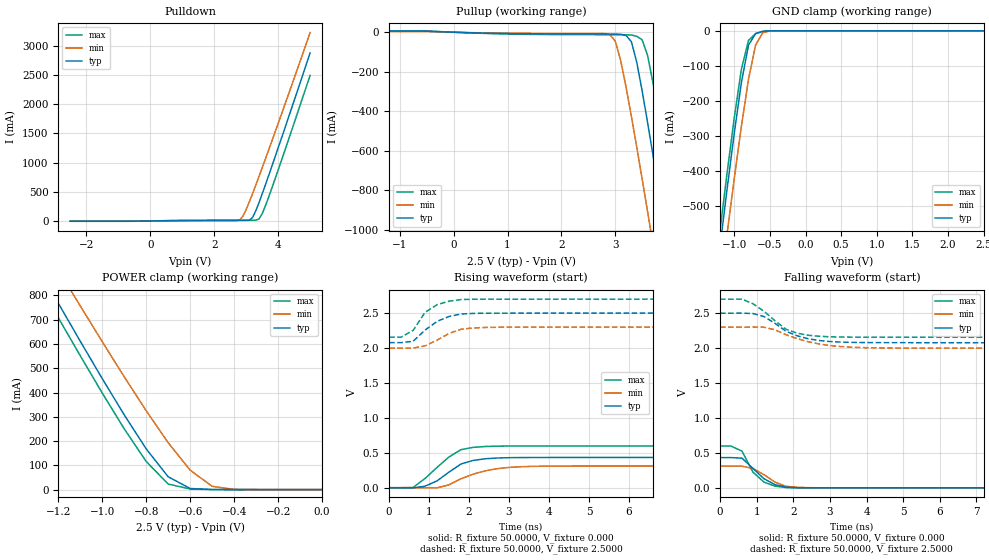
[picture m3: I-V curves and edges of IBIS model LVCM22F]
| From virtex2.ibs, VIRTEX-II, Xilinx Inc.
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|   Model LVCM22F
[Model]   LVCM22F
Model_type   I/O
Polarity   Non-Inverting
Enable   Active-Low
Vinh = 1.7V
Vinl = 0.7V
Vmeas =   1.2500V
Cref =  35.0000pF
Rref =   1.0000M
Vref =  0.000V
C_comp   7.0000pF   6.0000pF   8.0000pF
[Temperature Range]   25.0000   100.0000   0.000
[Voltage Range]   2.5000V   2.3000V   2.7000V
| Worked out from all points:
|   slope of the pulldown table from 0 to 0.375 V, typ, clamps not added: 122 ohm
|   slope of the pullup table from 0 to 0.375 V, typ, clamps not added: 116 ohm
|   GND clamp passes 1 mA (typ) near -0.57 V on its own axis
|   POWER clamp passes 1 mA (typ) near -0.52 V on its own axis
|   rising waveform, R_fixture 50.0000, V_fixture 0.000: 20-80 % time 684ps typ, 900ps min, 739ps max; typ from 0 V to 0.433 V
|   rising waveform, R_fixture 50.0000, V_fixture 2.5000: 20-80 % time 622ps typ, 653ps min, 505ps max; typ from 2.08 V to 2.5 V
|   falling waveform, R_fixture 50.0000, V_fixture 0.000: 20-80 % time 596ps typ, 605ps min, 475ps max; typ from 0.433 V to 0 V
|   falling waveform, R_fixture 50.0000, V_fixture 2.5000: 20-80 % time 896ps typ, 1.11ns min, 809ps max; typ from 2.5 V to 2.08 V
[Pulldown]
| voltage   I(typ)   I(min)   I(max)
-2.5V     -5.481mA   -3.66mA    -6.342mA
2.6V      8.571mA    6.23mA     11mA
2.8V      8.605mA    18.9mA     11.04mA
2.9V      8.633mA    83.75mA    11.06mA
3.1V      12.78mA    327.5mA    11.1mA
3.2V      58.36mA    467.2mA    11.32mA
3.3V      171.9mA    611.7mA    13.35mA
3.4V      311.3mA    758.9mA    31.74mA
3.5V      460.3mA    908mA      121.4mA
3.7V      770.7mA    1.209A     402.1mA
4V        1.249A     1.668A     870.2mA
5V        2.877A     3.226A     2.492A
[Pullup]
| voltage   I(typ)   I(min)   I(max)
-2.5V     5.869mA    3.31mA     7.396mA
2.9V      -9.073mA   -11.85mA   -12.55mA
3V        -9.217mA   -45.04mA   -12.6mA
3.1V      -10.44mA   -142mA     -12.65mA
3.3V      -47.69mA   -425.5mA   -14.17mA
3.4V      -152.4mA   -582.2mA   -20.41mA
3.5V      -297mA     -743mA     -38.14mA
3.6V      -455.4mA   -906.4mA   -116.8mA
3.8V      -788.3mA   -1.238A    -410.7mA
4V        -1.13A     -1.574A    -743.1mA
4.2V      -1.477A    -1.913A    -1.085A
5V        -2.884A    -3.282A    -2.488A
[GND_clamp]
| voltage   I(typ)   I(min)   I(max)
-2.5V     -2.881A    -2.936A    -2.838A
-1.2V     -617mA     -740.6mA   -570.6mA
-1.1V     -452.1mA   -579.7mA   -406.1mA
-1V       -293.4mA   -423mA     -249mA
-900mV    -148mA     -273.4mA   -110.1mA
-800mV    -41mA      -138.5mA   -27.22mA
-700mV    -7.569mA   -40.19mA   -8.128mA
-600mV    -1.403mA   -5.589mA   -1.597mA
-500mV    -127.6uA   -662.5uA   -122uA
2.5V      397.5nA    2.548uA    351.3nA
[POWER_clamp]
| voltage   I(typ)   I(min)   I(max)
-2.5V     2.874A     2.908A     2.816A
-1.3V     925.8mA    1.055A     866.1mA
-1.2V     767.5mA    905.5mA    707.7mA
-1.1V     610.9mA    756.3mA    551.2mA
-1V       456.9mA    609.1mA    397.6mA
-900mV    307.7mA    464.5mA    250.2mA
-800mV    167.5mA    324.6mA    115.6mA
-700mV    52.75mA    192.9mA    22.81mA
-600mV    4.571mA    79.88mA    2.444mA
-500mV    271.3uA    13.45mA    251.8uA
-400mV    16.93uA    820.9uA    15.04uA
0V        397.5nA    368nA      428.7nA
[Ramp]
| variable   typ   min   max
dV/dt_r   0.2598/0.7377n   0.1865/0.9257n   0.3590/0.6380n
dV/dt_f   0.2538/0.9437n   0.1806/1.1440n   0.3270/0.8292n
R_load = 50.0000
[Rising Waveform]
R_fixture = 50.0000
V_fixture = 0.000
| time   V(typ)   V(min)   V(max)
0s        14.97uV    15.8uV     15.19uV
600ps     -1.679mV   -36.34uV   3.043mV
900ps     22.16mV    -2.088mV   133.4mV
1.2ns     98.34mV    -1.759mV   291.9mV
1.5ns     224.7mV    41.66mV    441.5mV
1.8ns     340.1mV    128.2mV    545.6mV
2.4ns     414.5mV    241.2mV    590mV
3ns       429.9mV    290.8mV    596.7mV
3.9ns     432.8mV    308.3mV    598mV
15ns      433.1mV    310.8mV    598.4mV
[Rising Waveform]
R_fixture = 50.0000
V_fixture = 2.5000
V_fixture_min = 2.3000
V_fixture_max = 2.7000
| time   V(typ)   V(min)   V(max)
0s        2.077V     1.999V     2.155V
300ps     2.077V     1.999V     2.156V
600ps     2.096V     1.999V     2.253V
900ps     2.257V     2.031V     2.511V
1.2ns     2.382V     2.113V     2.621V
1.5ns     2.452V     2.209V     2.671V
1.8ns     2.487V     2.269V     2.694V
2.1ns     2.495V     2.287V     2.698V
3ns       2.499V     2.299V     2.7V
15ns      2.5V       2.3V       2.7V
[Falling Waveform]
R_fixture = 50.0000
V_fixture = 0.000
| time   V(typ)   V(min)   V(max)
0s        433.1mV    310.8mV    598.4mV
300ps     433.1mV    310.8mV    598.5mV
600ps     425.1mV    310.4mV    525.7mV
900ps     278.3mV    277.1mV    225.1mV
1.2ns     131mV      188.9mV    82.29mV
1.5ns     46.23mV    82.79mV    25.35mV
1.8ns     8.845mV    21.84mV    4.019mV
2.1ns     2.591mV    7.985mV    964.4uV
3ns       114.5uV    414.1uV    46.86uV
15ns      1.966uV    2.77uV     2.285uV
[Falling Waveform]
R_fixture = 50.0000
V_fixture = 2.5000
V_fixture_min = 2.3000
V_fixture_max = 2.7000
| time   V(typ)   V(min)   V(max)
0s        2.5V       2.3V       2.7V
600ps     2.501V     2.3V       2.701V
900ps     2.495V     2.302V     2.635V
1.2ns     2.452V     2.299V     2.528V
1.8ns     2.242V     2.192V     2.27V
2.1ns     2.177V     2.137V     2.215V
2.7ns     2.109V     2.059V     2.17V
3.3ns     2.087V     2.022V     2.159V
4.5ns     2.078V     2.002V     2.156V
15ns      2.077V     1.999V     2.155V
